| IBIS file stm32n657_vfbga264.ibs
[IBIS ver] 4.2
[File name] stm32n657_vfbga264.ibs
[File Rev] 1
[Date]  20-09-2024
[Source] Data Created at STMicroelectronics
[Notes]  File originated from ELDO simulations.
[Disclaimer]  This information is for modeling purpose only and is
   not guaranteed. The information is subject to change without
   notice.
[Copyright] Copyright 2024 STMicroelectronics Inc.
|   Component stm32n657_vfbga264
[Component] stm32n657_vfbga264
[Manufacturer] STMicroelectronics
[Package]
| variable   typ   min   max
R_pkg  0  NA  NA
L_pkg  0  NA  NA
C_pkg  0  NA  NA
[Pin]   signal_name   model_name
A1  PDR_ON  nc
A2  PQ6  io8_tt
A3  OTG2_HSDM  USB2_HS_IBIS
A4  VDD33USB  power
A5  OTG1_HSDM  USB2_HS_IBIS
A6  UCPD1_CC1  nc
A7  PH0-OSC_IN  isudq_tt
A8  PC10  io8_tt_i3c
A9  PC1  io8_tt_i3c
A10  PC4  io8_tt
A11  PE13  io8_tt_i3c
A12  PE15  io8_tt_i3c
A13  PD10  io8_tt
A14  PD1  io8_tt
A15  PE8  io8_tt
A16  PE9  io8_tt
A17  VSS  gnd
B1  PH3  io8_tt
B2  PH6  io8_tt
B3  OTG2_HSDP  USB2_HS_IBIS
B4  NC  nc
B5  OTG1_HSDP  USB2_HS_IBIS
B6  UCPD1_CC2  nc
B7  PH1-OSC_OUT  isudq_tt
B8  PC11  io8_tt_i3c
B9  PC6  io8_tt
B10  PC5  io8_tt
B11  PE14  io8_tt_i3c
B12  PE12  io8_tt
B13  PE7  io8_tt
B14  PD15  io8_tt_i3c
B15  PD4  io8_tt_i3c
B16  PE10  io8_tt
B17  PB14  io8_tt
C1  PC15-OSC32_OUT  io8_tt_sw
C2  PH8  io8_tt_i3c
C3  OTG1_ID  nc
C4  NC  nc
C5  VDDA18USB  power
C6  OTG1_TXRTUNE  nc
C7  PC9  io8_tt_i3c
C8  PC12  io8_tt
C9  PC7  io8_tt
C10  PC0  io8_tt
C11  PE5  io8_tt_i3c
C12  PD2  io8_tt
C13  PD12  io8_tt
C14  PD14  io8_tt_i3c
C15  PB13  io8_tt
C16  PB2  io8_tt
C17  PD13  io8_tt
D1  PC14-OSC32_IN  io8_tt_sw
D2  PH7  io8_tt_i3c
D3  PQ3  io8_tt
D4  PQ4  io8_tt
D5  PQ5  io8_tt
D6  OTG2_TXRTUNE  nc
D7  PC8  io8_tt_i3c
D8  PH9  io8_tt_i3c
D9  PC2  io8_tt
D10  PE4  io8_tt
D11  PE6  io8_tt_i3c
D12  PD6  io8_tt
D13  PD0  io8_tt
D14  PD5  io8_tt
D15  PB9  io8_tt
D16  PB8  io8_tt
D17  PB15  io8_tt
E1  VBAT  power
E2  PWR_ON  io8_tt
E3  PQ2  io8_tt
E4  PQ1  io8_tt
E5  PQ0  io8_tt
E6  OTG2_ID  nc
E7  PH2  io8_tt
E8  VDDIO4  power
E9  VDDIO5  power
E10  PC3  io8_tt
E11  PE11  io8_tt
E12  PD7  io8_tt
E13  PD3  io8_tt_i3c
E14  PD8  io8_tt
E15  PB0  io8_tt
E16  PB7  io8_tt
E17  PB6  io8_tt
F1  V08CAP  nc
F2  VSSAPMU  nc
F3  PC13  io8_tt_tamp
F4  PH4  io8_tt
F5  PH5  io8_tt
F6  VDDA18AON  nc
F7  VSS  gnd
F8  VDDIO4  power
F9  VDDIO5  power
F10  VSS  gnd
F11  VSS  gnd
F12  VSS  gnd
F13  PB3  io8_tt
F14  PE3  io8_tt
F15  PE2  io8_tt
F16  PE0  io8_tt
F17  PE1  io8_tt
G1  VDDA18PMU  nc
G2  VFBSMPS  nc
G3  NRST  ioreset_tt_v18
G4  BOOT0  isudq_tt
G5  PQ7  io8_tt_tamp
G6  VSSAON  nc
G12  VSS  gnd
G13  VDD  power
G14  PD11  io8_tt_i3c
G15  PP7  io8_tt
G16  PP6  io8_tt
G17  PP0  io8_tt
H1  VSSSMPS  nc
H2  VSSSMPS  nc
H3  VSSSMPS  nc
H4  VSSSMPS  nc
H5  VSSSMPS  nc
H6  VSSSMPS  nc
H12  VDD  power
H13  VDD  power
H14  PD9  io8_tt
H15  PP4  io8_tt
H16  PP1  io8_tt
H17  PP15  io8_tt
J1  VLXSMPS  nc
J2  VLXSMPS  nc
J3  VLXSMPS  nc
J4  VLXSMPS  nc
J5  VLXSMPS  nc
J6  VLXSMPS  nc
J12  VDD  power
J13  VDD  power
J14  PP5  io8_tt
J15  PP12  io8_tt
J16  PP3  io8_tt
J17  PP2  io8_tt
K1  VDDSMPS  nc
K2  VDDSMPS  nc
K3  VDDSMPS  nc
K4  VDDSMPS  nc
K5  VDDSMPS  nc
K6  VDDSMPS  nc
K12  VSS  gnd
K13  VDD  power
K14  PP13  io8_tt
K15  PO5  io8_tt
K16  PO1  io8_tt
K17  PO2  io8_tt
L1  PG7  io8_tt
L2  PF4  io8_tt
L3  PG6  io8_tt
L4  PF10  io8_tt
L5  PF6  io8_tt
L6  VDDCORE  nc
L12  VDDCORE  nc
L13  VDDIO2  power
L14  VDDIO2  power
L15  PP11  io8_tt
L16  PP8  io8_tt
L17  PP14  io8_tt
M1  PF7  io8_tt
M2  PF3  io8_tt
M3  PF5  io8_tt
M4  PG5  io8_tt
M5  VDDA18PLL  nc
M6  VSSA  nc
M7  VDDCORE  nc
M8  VSS  gnd
M9  VDDCORE  nc
M10  VSS  gnd
M11  VDDCORE  nc
M12  VSS  gnd
M13  VSS  gnd
M14  VDDIO2  power
M15  VDDIO2  power
M16  PO3  io8_tt
M17  PO0  io8_tt
N1  PF15  io8_tt
N2  PF14  io8_tt
N3  PF8  io8_tt
N4  PF2  io8_tt
N5  VSS  gnd
N6  VDDA18ADC  nc
N7  VSS  gnd
N8  VDDCORE  nc
N9  VSS  gnd
N10  VDDCORE  nc
N11  VSS  gnd
N12  VDDCORE  nc
N13  VDDIO3  power
N14  PP9  io8_tt
N15  PP10  io8_tt
N16  PO4  io8_tt
N17  PN4  io8_tt
P1  PF9  io8_tt
P2  PG4  io8_tt
P3  PF11  io8_tt
P4  PF1  io8_tt
P5  CSI_REXT  nc
P6  PG14  io8_tt
P7  PA9  io8_tt_i3c
P8  PA6  io8_tt_i3c
P9  PA1  io8_tt
P10  PB11  io8_tt_i3c
P11  VDDCORE  nc
P12  PA15  io8_tt
P13  VDDIO3  power
P14  PN12  io8_tt
P15  PN6  io8_tt
P16  PN8  io8_tt
P17  PN0  io8_tt
R1  PG3  io8_tt
R2  PF13  io8_tt
R3  PF0  io8_tt
R4  VDDCSI  nc
R5  VDDA18CSI  power
R6  PG15  io8_tt
R7  PA10  io8_tt
R8  PA5  io8_tt_i3c
R9  PG1  io8_tt
R10  PB12  io8_tt_i3c
R11  PB1  io8_tt
R12  PA7  io8_tt
R13  PG0  io8_tt
R14  PA3  io8_tt
R15  PN3  io8_tt
R16  PN5  io8_tt
R17  PN1  io8_tt
T1  PF12  io8_tt
T2  VREFM  nc
T3  CSI_CKP  DPHY_IBIS_L1
T4  CSI_D1P  DPHY_IBIS_L1
T5  CSI_D0P  DPHY_IBIS_L1
T6  PA14  io8_tt
T7  PA11  io8_tt
T8  PA2  io8_tt
T9  PG12  io8_tt
T10  PG10  io8_tt
T11  PG2  io8_tt
T12  PB4  io8_tt
T13  PG9  io8_tt
T14  PG8  io8_tt
T15  PN9  io8_tt
T16  PN7  io8_tt
T17  PN2  io8_tt
U1  VSS  gnd
U2  VREFP  nc
U3  CSI_CKN  DPHY_IBIS_L1
U4  CSI_D1N  DPHY_IBIS_L1
U5  CSI_D0N  DPHY_IBIS_L1
U6  PA13  io8_tt
U7  PA12  io8_tt
U8  PA8  io8_tt_i3c
U9  PG13  io8_tt
U10  PA0  io8_tt
U11  PB10  io8_tt_i3c
U12  PB5  io8_tt_i3c
U13  PG11  io8_tt
U14  PA4  io8_tt
U15  PN10  io8_tt
U16  PN11  io8_tt
U17  VSS  gnd
[Package Model]   486-bga-14x14mm-264-220805
[Pin Mapping]   pulldown_ref   pullup_ref   | Comment
A1  nc  nc
A2  gnd  VDD
A3  gnd  VDD33USB
A4  nc  VDD33USB
A5  gnd  VDD33USB
A6  nc   nc
A7  gnd  VDD
A8  gnd  VDDIO4
A9  gnd  VDDIO4
A10  gnd  VDDIO5
A11  gnd  VDD
A12  gnd  VDD
A13  gnd  VDD
A14  gnd  VDD
A15  gnd  VDD
A16  gnd  VDD
A17  gnd  nc
B1  gnd  VDD
B2  gnd  VDD
B3  gnd  VDD33USB
B4  nc   nc
B5  gnd  VDD33USB
B6  nc   nc
B7  gnd  VDD
B8  gnd  VDDIO4
B9  gnd  VDDIO4
B10  gnd  VDDIO5
B11  gnd  VDD
B12  gnd  VDD
B13  gnd  VDD
B14  gnd  VDD
B15  gnd  VDD
B16  gnd  VDD
B17  gnd  VDD
C1  gnd  VSW
C2  gnd  VDD
C3  nc   nc
C4  nc   nc
C5  nc  VDDA18USB
C6  nc   nc
C7  gnd  VDDIO4
C8  gnd  VDDIO4
C9  gnd  VDDIO4
C10  gnd  VDDIO5
C11  gnd  VDD
C12  gnd  VDD
C13  gnd  VDD
C14  gnd  VDD
C15  gnd  VDD
C16  gnd  VDD
C17  gnd  VDD
D1  gnd  VSW
D2  gnd  VDD
D3  gnd  VDD
D4  gnd  VDD
D5  gnd  VDD
D6  nc   nc
D7  gnd  VDDIO4
D8  gnd  VDDIO4
D9  gnd  VDDIO5
D10  gnd  VDDIO5
D11  gnd  VDD
D12  gnd  VDD
D13  gnd  VDD
D14  gnd  VDD
D15  gnd  VDD
D16  gnd  VDD
D17  gnd  VDD
E1  nc  VSW
E2  gnd  VDD
E3  gnd  VDD
E4  gnd  VDD
E5  gnd  VDD
E6  nc   nc
E7  gnd  VDDIO4
E8  nc  VDDIO4
E9  nc  VDDIO5
E10  gnd  VDDIO5
E11  gnd  VDD
E12  gnd  VDD
E13  gnd  VDD
E14  gnd  VDD
E15  gnd  VDD
E16  gnd  VDD
E17  gnd  VDD
F1  nc  nc
F2  nc  nc
F3  gnd  VSW
F4  gnd  VDD
F5  gnd  VDD
F6  nc  nc
F7  gnd  nc
F8  nc  VDDIO4
F9  nc  VDDIO5
F10  gnd  nc
F11  gnd  nc
F12  gnd  nc
F13  gnd  VDD
F14  gnd  VDD
F15  gnd  VDD
F16  gnd  VDD
F17  gnd  VDD
G1  nc  nc
G2  nc  nc
G3  gnd  VDD
G4  gnd  VDD
G5  gnd  VSW
G6  nc  nc
G12  gnd  nc
G13  nc  VDD
G14  gnd  VDD
G15  gnd  VDDIO2
G16  gnd  VDDIO2
G17  gnd  VDDIO2
H1  nc  nc
H2  nc  nc
H3  nc  nc
H4  nc  nc
H5  nc  nc
H6  nc  nc
H12  nc  VDD
H13  nc  VDD
H14  gnd  VDD
H15  gnd  VDDIO2
H16  gnd  VDDIO2
H17  gnd  VDDIO2
J1  nc  nc
J2  nc  nc
J3  nc  nc
J4  nc  nc
J5  nc  nc
J6  nc  nc
J12  nc  VDD
J13  nc  VDD
J14  gnd  VDDIO2
J15  gnd  VDDIO2
J16  gnd  VDDIO2
J17  gnd  VDDIO2
K1  nc  nc
K2  nc  nc
K3  nc  nc
K4  nc  nc
K5  nc  nc
K6  nc  nc
K12  gnd  nc
K13  nc  VDD
K14  gnd  VDDIO2
K15  gnd  VDDIO2
K16  gnd  VDDIO2
K17  gnd  VDDIO2
L1  gnd  VDD
L2  gnd  VDD
L3  gnd  VDD
L4  gnd  VDD
L5  gnd  VDD
L6  nc  nc
L12  nc  nc
L13  nc  VDDIO2
L14  nc  VDDIO2
L15  gnd  VDDIO2
L16  gnd  VDDIO2
L17  gnd  VDDIO2
M1  gnd  VDD
M2  gnd  VDD
M3  gnd  VDD
M4  gnd  VDD
M5  nc  nc
M6  nc  nc
M7  nc  nc
M8  gnd  nc
M9  nc  nc
M10  gnd  nc
M11  nc  nc
M12  gnd  nc
M13  gnd  nc
M14  nc  VDDIO2
M15  nc  VDDIO2
M16  gnd  VDDIO2
M17  gnd  VDDIO2
N1  gnd  VDD
N2  gnd  VDD
N3  gnd  VDD
N4  gnd  VDD
N5  gnd  nc
N6  nc  nc
N7  gnd  nc
N8  nc  nc
N9  gnd  nc
N10  nc  nc
N11  gnd  nc
N12  nc  nc
N13  nc  VDDIO3
N14  gnd  VDDIO2
N15  gnd  VDDIO2
N16  gnd  VDDIO2
N17  gnd  VDDIO3
P1  gnd  VDD
P2  gnd  VDD
P3  gnd  VDD
P4  gnd  VDD
P5  nc   nc
P6  gnd  VDD
P7  gnd  VDD
P8  gnd  VDD
P9  gnd  VDD
P10  gnd  VDD
P11  nc  nc
P12  gnd  VDD
P13  nc  VDDIO3
P14  gnd  VDDIO3
P15  gnd  VDDIO3
P16  gnd  VDDIO3
P17  gnd  VDDIO3
R1  gnd  VDD
R2  gnd  VDD
R3  gnd  VDD
R4  nc  nc
R5  nc  VDDA18CSI
R6  gnd  VDD
R7  gnd  VDD
R8  gnd  VDD
R9  gnd  VDD
R10  gnd  VDD
R11  gnd  VDD
R12  gnd  VDD
R13  gnd  VDD
R14  gnd  VDD
R15  gnd  VDDIO3
R16  gnd  VDDIO3
R17  gnd  VDDIO3
T1  gnd  VDD
T2  nc  nc
T3  gnd  VDDA18CSI
T4  gnd  VDDA18CSI
T5  gnd  VDDA18CSI
T6  gnd  VDD
T7  gnd  VDD
T8  gnd  VDD
T9  gnd  VDD
T10  gnd  VDD
T11  gnd  VDD
T12  gnd  VDD
T13  gnd  VDD
T14  gnd  VDD
T15  gnd  VDDIO3
T16  gnd  VDDIO3
T17  gnd  VDDIO3
U1  gnd  nc
U2  nc  nc
U3  gnd  VDDA18CSI
U4  gnd  VDDA18CSI
U5  gnd  VDDA18CSI
U6  gnd  VDD
U7  gnd  VDD
U8  gnd  VDD
U9  gnd  VDD
U10  gnd  VDD
U11  gnd  VDD
U12  gnd  VDD
U13  gnd  VDD
U14  gnd  VDD
U15  gnd  VDDIO3
U16  gnd  VDDIO3
U17  gnd  nc
[Diff_pin]   inv_pin   vdiff   tdelay_typ   tdelay_min   tdelay_max
T5   U5   400mV   0ns   NA   NA
T4   U4   400mV   0ns   NA   NA
T3   U3   400mV   0ns   NA   NA
B5   A5   150mV   0ns   NA   NA
B3   A3   150mV   0ns   NA   NA
[Model Selector] DPHY_IBIS_L1
DPHY_RX_2P5G_L1   DPHY HSRX model at 2.5Gbps for lane 1
DPHY_RX_1P5G_L1   DPHY HSRX model at 1.5Gbps for lane 1
[Model Selector] USB2_HS_IBIS
USB2_HSRX   USB2 HSRX model
USB2_HSTX_00_0_01_0011_11   TuningBits_AMP_PULSE_RISE_REF_XV=00_0_01_0011_11
USB2_HSTX_00_0_10_0101_11   TuningBits_AMP_PULSE_RISE_REF_XV=00_0_10_0101_11
USB2_HSTX_00_0_11_0111_11   TuningBits_AMP_PULSE_RISE_REF_XV=00_0_11_0111_11
USB2_HSTX_00_1_01_0011_11   TuningBits_AMP_PULSE_RISE_REF_XV=00_1_01_0011_11
USB2_HSTX_00_1_10_0101_11   TuningBits_AMP_PULSE_RISE_REF_XV=00_1_10_0101_11
USB2_HSTX_00_1_11_0111_11   TuningBits_AMP_PULSE_RISE_REF_XV=00_1_11_0111_11
USB2_HSTX_01_0_01_0011_11   TuningBits_AMP_PULSE_RISE_REF_XV=01_0_01_0011_11
USB2_HSTX_01_0_10_0101_11   TuningBits_AMP_PULSE_RISE_REF_XV=01_0_10_0101_11
USB2_HSTX_01_0_11_0111_11   TuningBits_AMP_PULSE_RISE_REF_XV=01_0_11_0111_11
USB2_HSTX_01_1_01_0011_11   TuningBits_AMP_PULSE_RISE_REF_XV=01_1_01_0011_11
USB2_HSTX_01_1_10_0101_11   TuningBits_AMP_PULSE_RISE_REF_XV=01_1_10_0101_11
USB2_HSTX_01_1_11_0111_11   TuningBits_AMP_PULSE_RISE_REF_XV=01_1_11_0111_11
USB2_HSTX_10_0_01_0011_11   TuningBits_AMP_PULSE_RISE_REF_XV=10_0_01_0011_11
USB2_HSTX_10_0_10_0101_11   TuningBits_AMP_PULSE_RISE_REF_XV=10_0_10_0101_11
USB2_HSTX_10_0_11_0111_11   TuningBits_AMP_PULSE_RISE_REF_XV=10_0_11_0111_11
USB2_HSTX_10_1_01_0011_11   TuningBits_AMP_PULSE_RISE_REF_XV=10_1_01_0011_11
USB2_HSTX_10_1_10_0101_11   TuningBits_AMP_PULSE_RISE_REF_XV=10_1_10_0101_11
USB2_HSTX_10_1_11_0111_11   TuningBits_AMP_PULSE_RISE_REF_XV=10_1_11_0111_11
[Model Selector] io8_tt
io8_tt_ls_3v3   "GPIO - 3V tolerant - 3.3V range - Low speed"
io8_tt_ms_3v3   "GPIO - 3V tolerant - 3.3V range - Med speed"
io8_tt_fs_3v3   "GPIO - 3V tolerant - 3.3V range - Fast speed"
io8_tt_hs_3v3   "GPIO - 3V tolerant - 3.3V range - High speed"
io8_tt_hslv_ls_1v8   "GPIO HSLV - 3V tolerant - 1.8V range - Low speed"
io8_tt_hslv_ms_1v8   "GPIO HSLV - 3V tolerant - 1.8V range - Med speed"
io8_tt_hslv_fs_1v8   "GPIO HSLV - 3V tolerant - 1.8V range - Fast speed"
io8_tt_hslv_hs_1v8   "GPIO HSLV - 3V tolerant - 1.8V range - High speed"
[Model Selector] io8_tt_i3c
io8_tt_ls_3v3   "GPIO - 3V tolerant - 3.3V range - Low speed"
io8_tt_ms_3v3   "GPIO - 3V tolerant - 3.3V range - Med speed"
io8_tt_fs_3v3   "GPIO - 3V tolerant - 3.3V range - Fast speed"
io8_tt_hs_3v3   "GPIO - 3V tolerant - 3.3V range - High speed"
io8_tt_hslv_ls_1v8   "GPIO HSLV - 3V tolerant - 1.8V range - Low speed"
io8_tt_hslv_ms_1v8   "GPIO HSLV - 3V tolerant - 1.8V range - Med speed"
io8_tt_hslv_fs_1v8   "GPIO HSLV - 3V tolerant - 1.8V range - Fast speed"
io8_tt_hslv_hs_1v8   "GPIO HSLV - 3V tolerant - 1.8V range - High speed"
io8_tt_i3c_3v3   "GPIO - 3V tolerant - 3.3V range - Open drain"
[Model Selector] io8_tt_tamp
io8_tt_ls_3v3   "GPIO - 3V tolerant - 3.3V range - Low speed"
io8_tt_ms_3v3   "GPIO - 3V tolerant - 3.3V range - Med speed"
io8_tt_fs_3v3   "GPIO - 3V tolerant - 3.3V range - Fast speed"
io8_tt_hs_3v3   "GPIO - 3V tolerant - 3.3V range - High speed"
io8_tt_hslv_ls_1v8   "GPIO HSLV - 3V tolerant - 1.8V range - Low speed"
io8_tt_hslv_ms_1v8   "GPIO HSLV - 3V tolerant - 1.8V range - Med speed"
io8_tt_hslv_fs_1v8   "GPIO HSLV - 3V tolerant - 1.8V range - Fast speed"
io8_tt_hslv_hs_1v8   "GPIO HSLV - 3V tolerant - 1.8V range - High speed"
io8_tt_tamp_1v8   "GPIO TAMP - 3V tolerant - 1.8V range - Open drain"
io8_tt_tamp_3v3   "GPIO TAMP - 3V tolerant - 3.3V range - Open drain"
[Model Selector] io8_tt_sw
io8_tt_sw_1v8   "GPIO SW - 3V tolerant - 1.8V range"
io8_tt_sw_3v3   "GPIO SW - 3V tolerant - 3.3V range"
[Model Selector] ioreset_tt_v18
ioreset_tt_v18_1v8   "Reset PAD. 3V tolerant. 1.8V range"
ioreset_tt_v18_3v3   "Reset PAD. 3V tolerant. 3.3V range"
[Model Selector] isudq_tt
isudq_tt_1v8   "Input Buffer - 3V tolerant - 1.8V range"
isudq_tt_3v3   "Input Buffer - 3V tolerant - 3.3V range"
[Define Package Model]  486-bga-14x14mm-264-220805
[Manufacturer]  unknown
[OEM]  unknown
[Description]  unknown
[Number Of Pins]  214
[Pin Numbers]
G4 | BOOT0
U3 | CSI_CKN
T3 | CSI_CKP
U5 | CSI_D0N
T5 | CSI_D0P
U4 | CSI_D1N
T4 | CSI_D1P
P5 | CSI_REXT
G3 | NRST
A5 | OTG1_HSDM
B5 | OTG1_HSDP
C3 | OTG1_ID
C6 | OTG1_TXRTUNE
B4 | NC
A3 | OTG2_HSDM
B3 | OTG2_HSDP
E6 | OTG2_ID
D6 | OTG2_TXRTUNE
C4 | NC
U10 | PA0
P9 | PA1
T8 | PA2
R14 | PA3
U14 | PA4
R8 | PA5
P8 | PA6
R12 | PA7
U8 | PA8
P7 | PA9
R7 | PA10
T7 | PA11
U7 | PA12
U6 | PA13
T6 | PA14
P12 | PA15
E15 | PB0
R11 | PB1
C16 | PB2
F13 | PB3
T12 | PB4
U12 | PB5
E17 | PB6
E16 | PB7
D16 | PB8
D15 | PB9
U11 | PB10
P10 | PB11
R10 | PB12
C15 | PB13
B17 | PB14
D17 | PB15
C10 | PC0
A9 | PC1
D9 | PC2
E10 | PC3
A10 | PC4
B10 | PC5
B9 | PC6
C9 | PC7
D7 | PC8
C7 | PC9
A8 | PC10
B8 | PC11
C8 | PC12
F3 | PC13
D1 | PC14-OSC32_IN
C1 | PC15-OSC32_OUT
D13 | PD0
A14 | PD1
C12 | PD2
E13 | PD3
B15 | PD4
D14 | PD5
D12 | PD6
E12 | PD7
E14 | PD8
H14 | PD9
A13 | PD10
G14 | PD11
C13 | PD12
C17 | PD13
C14 | PD14
B14 | PD15
A1 | PDR_ON
F16 | PE0
F17 | PE1
F15 | PE2
F14 | PE3
D10 | PE4
C11 | PE5
D11 | PE6
B13 | PE7
A15 | PE8
A16 | PE9
B16 | PE10
E11 | PE11
B12 | PE12
A11 | PE13
B11 | PE14
A12 | PE15
R3 | PF0
P4 | PF1
N4 | PF2
M2 | PF3
L2 | PF4
M3 | PF5
L5 | PF6
M1 | PF7
N3 | PF8
P1 | PF9
L4 | PF10
P3 | PF11
T1 | PF12
R2 | PF13
N2 | PF14
N1 | PF15
R13 | PG0
R9 | PG1
T11 | PG2
R1 | PG3
P2 | PG4
M4 | PG5
L3 | PG6
L1 | PG7
T14 | PG8
T13 | PG9
T10 | PG10
U13 | PG11
T9 | PG12
U9 | PG13
P6 | PG14
R6 | PG15
A7 | PH0-OSC_IN
B7 | PH1-OSC_OUT
E7 | PH2
B1 | PH3
F4 | PH4
F5 | PH5
B2 | PH6
D2 | PH7
C2 | PH8
D8 | PH9
P17 | PN0
R17 | PN1
T17 | PN2
R15 | PN3
N17 | PN4
R16 | PN5
P15 | PN6
T16 | PN7
P16 | PN8
T15 | PN9
U15 | PN10
U16 | PN11
P14 | PN12
M17 | PO0
K16 | PO1
K17 | PO2
M16 | PO3
N16 | PO4
K15 | PO5
G17 | PP0
H16 | PP1
J17 | PP2
J16 | PP3
H15 | PP4
J14 | PP5
G16 | PP6
G15 | PP7
L16 | PP8
N14 | PP9
N15 | PP10
L15 | PP11
J15 | PP12
K14 | PP13
L17 | PP14
H17 | PP15
E5 | PQ0
E4 | PQ1
E3 | PQ2
D3 | PQ3
D4 | PQ4
D5 | PQ5
A2 | PQ6
G5 | PQ7
E2 | PWR_ON
A6 | UCPD1_CC1
B6 | UCPD1_CC2
F1 | V08CAP
E1 | VBAT
A4 | VDD33USB
G13 | VDD
N6 | VDDA18ADC
F6 | VDDA18AON
R5 | VDDA18CSI
M5 | VDDA18PLL
G1 | VDDA18PMU
C5 | VDDA18USB
L6 | VDDCORE
R4 | VDDCSI
L13 | VDDIO2
N13 | VDDIO3
E8 | VDDIO4
E9 | VDDIO5
K1 | VDDSMPS
G2 | VFBSMPS
J1 | VLXSMPS
T2 | VREFM
U2 | VREFP
A17 | VSS
M6 | VSSA
G6 | VSSAON
F2 | VSSAPMU
H1 | VSSSMPS
|[Merged Pins]  G13
|H12  |  VDD
|H13  |  VDD
|J12  |  VDD
|J13  |  VDD
|K13  |  VDD
|[Merged Pins]  L6
|L12  |  VDDCORE
|M7  |  VDDCORE
|M9  |  VDDCORE
|M11  |  VDDCORE
|N8  |  VDDCORE
|N10  |  VDDCORE
|N12  |  VDDCORE
|P11  |  VDDCORE
|[Merged Pins]  L13
|L14  |  VDDIO2
|M14  |  VDDIO2
|M15  |  VDDIO2
|[Merged Pins]  N13
|P13  |  VDDIO3
|[Merged Pins]  E8
|F8  |  VDDIO4
|[Merged Pins]  E9
|F9  |  VDDIO5
|[Merged Pins]  K1
|K2  |  VDDSMPS
|K3  |  VDDSMPS
|K4  |  VDDSMPS
|K5  |  VDDSMPS
|K6  |  VDDSMPS
|[Merged Pins]  J1
|J2  |  VLXSMPS
|J3  |  VLXSMPS
|J4  |  VLXSMPS
|J5  |  VLXSMPS
|J6  |  VLXSMPS
|[Merged Pins]  A17
|F7  |  VSS
|F10  |  VSS
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[Model Data]
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[End Model Data]
[End Package Model]
| Models and submodels in the file (38): DPHY_RX_2P5G_L1 (Input), DPHY_RX_1P5G_L1 (Input), USB2_HSRX (Input), USB2_HSTX_00_0_01_0011_11 (Output), USB2_HSTX_00_0_10_0101_11 (Output), USB2_HSTX_00_0_11_0111_11 (Output), USB2_HSTX_00_1_01_0011_11 (Output), USB2_HSTX_00_1_10_0101_11 (Output), USB2_HSTX_00_1_11_0111_11 (Output), USB2_HSTX_01_0_01_0011_11 (Output), USB2_HSTX_01_0_10_0101_11 (Output), USB2_HSTX_01_0_11_0111_11 (Output), USB2_HSTX_01_1_01_0011_11 (Output), USB2_HSTX_01_1_10_0101_11 (Output), USB2_HSTX_01_1_11_0111_11 (Output), USB2_HSTX_10_0_01_0011_11 (Output), USB2_HSTX_10_0_10_0101_11 (Output), USB2_HSTX_10_0_11_0111_11 (Output), USB2_HSTX_10_1_01_0011_11 (Output), USB2_HSTX_10_1_10_0101_11 (Output), USB2_HSTX_10_1_11_0111_11 (Output), io8_tt_hslv_ls_1v8 (I/O), io8_tt_hslv_ms_1v8 (I/O), io8_tt_hslv_hs_1v8 (I/O), io8_tt_hslv_fs_1v8 (I/O), io8_tt_sw_1v8 (I/O), isudq_tt_1v8 (Input), io8_tt_tamp_1v8 (I/O), ioreset_tt_v18_1v8 (I/O_open_drain), io8_tt_ls_3v3 (I/O), io8_tt_ms_3v3 (I/O), io8_tt_hs_3v3 (I/O), io8_tt_fs_3v3 (I/O), io8_tt_sw_3v3 (I/O), io8_tt_i3c_3v3 (I/O_open_drain), isudq_tt_3v3 (Input), io8_tt_tamp_3v3 (I/O), ioreset_tt_v18_3v3 (I/O_open_drain)
